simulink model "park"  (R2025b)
settings: Solver=FixedStepAuto  StartTime=0.0  StopTime=10.0  FixedStep=1e-4  RelTol=1e-3
undefined symbols (not defined in the file): DiscIntNeverNeededParam

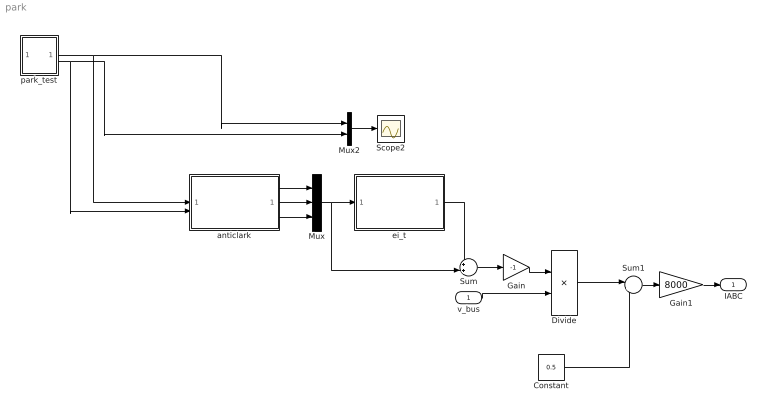
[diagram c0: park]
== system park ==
  v_bus : Inport
  Constant : Constant  Value=0.5
  Divide : Product  Inputs=*/
  Gain : Gain  Gain=-1
  Gain1 : Gain  Gain=8000
  Mux : Mux  Inputs=3
  Mux2 : Mux  Inputs=2
  Scope2 : Scope
  Sum : Sum  Inputs=++|
  Sum1 : Sum  Inputs=|++
  anticlark : Subsystem
  ei_t : Subsystem
  park_test : Subsystem
  IABC : Outport
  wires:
  Mux2/1 -> Scope2/1
  park_test/1(ualpha) -> anticlark/1(Valpha), Mux2/1
  park_test/2(ubeta) -> anticlark/2(Vbeta), Mux2/2
  anticlark/1(Va) -> Mux/1
  anticlark/2(Vb) -> Mux/2
  anticlark/3(Vc) -> Mux/3
  Mux/1 -> Sum/2, ei_t/1(Vabc)
  ei_t/1(ei_t1) -> Sum/1
  Sum/1 -> Gain/1
  Sum1/1 -> Gain1/1
  Gain1/1 -> IABC/1
  Gain/1 -> Divide/1
  v_bus/1 -> Divide/2
  Divide/1 -> Sum1/1
  Constant/1 -> Sum1/2

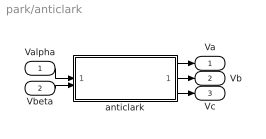
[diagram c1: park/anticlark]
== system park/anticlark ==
  Valpha : Inport
  Vbeta : Inport  Port=2
  anticlark : Subsystem
  Va : Outport
  Vb : Outport  Port=2
  Vc : Outport  Port=3
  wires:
  anticlark/3(Vc) -> Vc/1
  Vbeta/1 -> anticlark/2(Vbeta)
  anticlark/1(Va) -> Va/1
  anticlark/2(Vb) -> Vb/1
  Valpha/1 -> anticlark/1(Valpha)

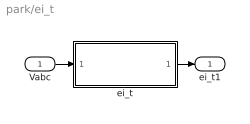
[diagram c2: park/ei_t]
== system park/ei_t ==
  Vabc : Inport
  ei_t : Subsystem
  ei_t1 : Outport
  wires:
  Vabc/1 -> ei_t/1(Vabc)
  ei_t/1(ei_t) -> ei_t1/1

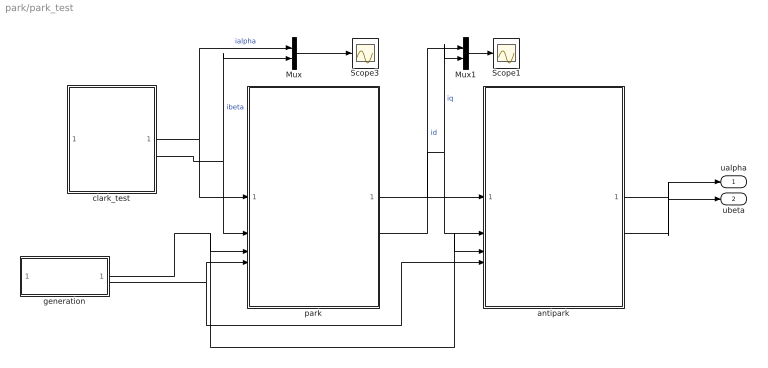
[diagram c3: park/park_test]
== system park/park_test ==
  Mux : Mux  Inputs=2
  Mux1 : Mux  Inputs=2
  Scope1 : Scope
  Scope3 : Scope
  antipark : Subsystem
  clark_test : Subsystem  TreatAsAtomicUnit=on
  generation : Subsystem
  park : Subsystem
  ualpha : Outport
  ubeta : Outport  Port=2
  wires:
  generation/2(cos) -> antipark/4(theta_cos), park/4(theta_cos)
  park/1(id) -> Mux1/1, antipark/1(ud)  "id"
  clark_test/1(ialpha) -> Mux/1, park/1(ialpha)  "ialpha"
  Mux1/1 -> Scope1/1
  clark_test/2(ibeta) -> Mux/2, park/2(ibeta)  "ibeta"
  generation/1(sin) -> antipark/3(theta_sin), park/3(theta_sin)
  park/2(iq) -> Mux1/2, antipark/2(uq)  "iq"
  Mux/1 -> Scope3/1
  antipark/2(ubeta) -> ubeta/1
  antipark/1(ualpha) -> ualpha/1

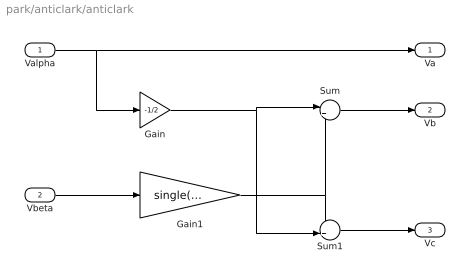
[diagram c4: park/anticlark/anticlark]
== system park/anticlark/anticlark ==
  Valpha : Inport
  Vbeta : Inport  Port=2
  Gain : Gain  Gain=-1/2
  Gain1 : Gain  Gain=single(sqrt(3)/2)
  Sum : Sum  Inputs=|++
  Sum1 : Sum  Inputs=-+|
  Va : Outport
  Vb : Outport  Port=2
  Vc : Outport  Port=3
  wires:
  Valpha/1 -> Gain/1, Va/1
  Gain/1 -> Sum1/2, Sum/1
  Gain1/1 -> Sum1/1, Sum/2
  Sum/1 -> Vb/1
  Vbeta/1 -> Gain1/1
  Sum1/1 -> Vc/1

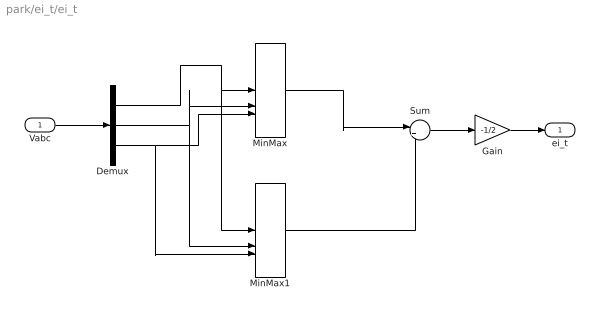
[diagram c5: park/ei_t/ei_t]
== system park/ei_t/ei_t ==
  Vabc : Inport
  Demux : Demux  Outputs=3
  Gain : Gain  Gain=-1/2
  MinMax : MinMax  Inputs=3
  MinMax1 : MinMax  Function=max  Inputs=3
  Sum : Sum  Inputs=|++
  ei_t : Outport
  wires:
  Vabc/1 -> Demux/1
  Demux/1 -> MinMax1/1, MinMax/1
  Demux/2 -> MinMax1/2, MinMax/2
  Demux/3 -> MinMax1/3, MinMax/3
  MinMax/1 -> Sum/1
  MinMax1/1 -> Sum/2
  Sum/1 -> Gain/1
  Gain/1 -> ei_t/1

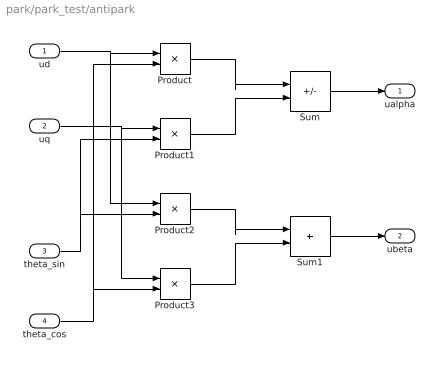
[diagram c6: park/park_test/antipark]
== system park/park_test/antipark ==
  ud : Inport
  uq : Inport  Port=2
  theta_sin : Inport  Port=3
  theta_cos : Inport  Port=4
  Product{,1..3} (4 alike) : Product
  Sum : Sum  Inputs=|+-
  Sum1 : Sum  Inputs=|++
  ualpha : Outport
  ubeta : Outport  Port=2
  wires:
  theta_cos/1 -> Product3/2, Product/2
  theta_sin/1 -> Product1/2, Product2/2
  uq/1 -> Product3/1, Product1/1
  ud/1 -> Product2/1, Product/1
  Product/1 -> Sum/1
  Product1/1 -> Sum/2
  Product2/1 -> Sum1/1
  Product3/1 -> Sum1/2
  Sum/1 -> ualpha/1
  Sum1/1 -> ubeta/1

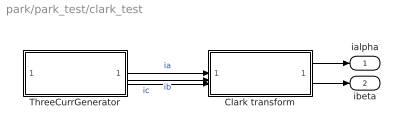
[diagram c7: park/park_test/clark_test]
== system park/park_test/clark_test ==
  Clark transform : Subsystem
  ThreeCurrGenerator : Subsystem
  ialpha : Outport
  ibeta : Outport  Port=2
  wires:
  Clark transform/1(ialpha) -> ialpha/1
  Clark transform/2(ibeta) -> ibeta/1
  ThreeCurrGenerator/1(ia) -> Clark transform/1(ia)  "ia"
  ThreeCurrGenerator/2(ib) -> Clark transform/2(ib)  "ib"
  ThreeCurrGenerator/3(ic) -> Clark transform/3(ic)  "ic"

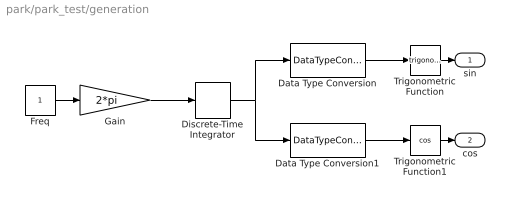
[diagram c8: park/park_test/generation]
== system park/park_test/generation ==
  Data Type Conversion : DataTypeConversion  OutDataTypeStr=single
  Data Type Conversion1 : DataTypeConversion  OutDataTypeStr=single
  Discrete-Time Integrator : DiscreteIntegrator  SampleTime=0.0001  ICPrevOutput=DiscIntNeverNeededParam  ICPrevScaledInput=DiscIntNeverNeededParam
  Freq : Constant
  Gain : Gain  Gain=2*pi
  Trigonometric Function : Trigonometry
  Trigonometric Function1 : Trigonometry  Operator=cos
  sin : Outport
  cos : Outport  Port=2
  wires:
  Freq/1 -> Gain/1
  Gain/1 -> Discrete-Time Integrator/1
  Discrete-Time Integrator/1 -> Data Type Conversion1/1, Data Type Conversion/1
  Data Type Conversion/1 -> Trigonometric Function/1
  Data Type Conversion1/1 -> Trigonometric Function1/1
  Trigonometric Function/1 -> sin/1
  Trigonometric Function1/1 -> cos/1

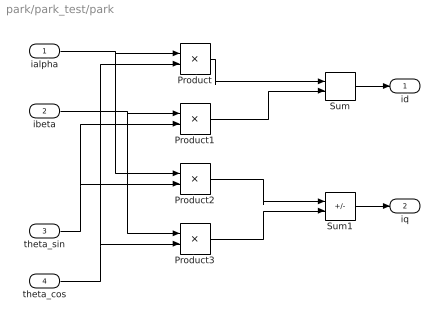
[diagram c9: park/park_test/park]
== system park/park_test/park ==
  ialpha : Inport
  ibeta : Inport  Port=2
  theta_sin : Inport  Port=3
  theta_cos : Inport  Port=4
  Product{,1..3} (4 alike) : Product
  Sum : Sum  Inputs=|++
  Sum1 : Sum  Inputs=|-+
  id : Outport
  iq : Outport  Port=2
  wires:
  ialpha/1 -> Product2/1, Product/1
  ibeta/1 -> Product1/1, Product3/1
  theta_sin/1 -> Product1/2, Product2/2
  theta_cos/1 -> Product3/2, Product/2
  Product/1 -> Sum/1
  Product1/1 -> Sum/2
  Product2/1 -> Sum1/1
  Product3/1 -> Sum1/2
  Sum1/1 -> iq/1
  Sum/1 -> id/1

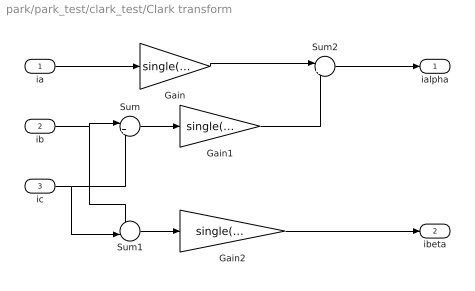
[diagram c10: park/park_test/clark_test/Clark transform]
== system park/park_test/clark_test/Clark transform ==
  ia : Inport
  ib : Inport  Port=2
  ic : Inport  Port=3
  Gain : Gain  Gain=single(2/3)
  Gain1 : Gain  Gain=single(1/3)
  Gain2 : Gain  Gain=single(sqrt(3)/3)
  Sum : Sum  Inputs=|++
  Sum1 : Sum  Inputs=+-|
  Sum2 : Sum  Inputs=|+-
  ialpha : Outport
  ibeta : Outport  Port=2
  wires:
  ia/1 -> Gain/1
  ib/1 -> Sum1/1, Sum/1
  ic/1 -> Sum1/2, Sum/2
  Sum/1 -> Gain1/1
  Sum1/1 -> Gain2/1
  Gain/1 -> Sum2/1
  Gain1/1 -> Sum2/2
  Gain2/1 -> ibeta/1
  Sum2/1 -> ialpha/1

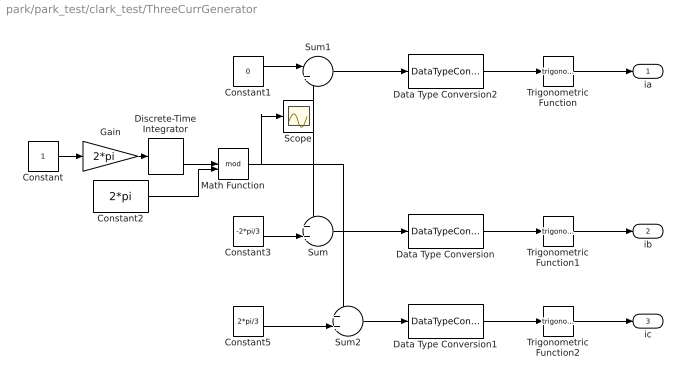
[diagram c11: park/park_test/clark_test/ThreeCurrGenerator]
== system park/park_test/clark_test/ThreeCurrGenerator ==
  Constant : Constant
  Constant1 : Constant  Value=0
  Constant2 : Constant  Value=2*pi
  Constant3 : Constant  Value=-2*pi/3
  Constant5 : Constant  Value=2*pi/3
  Data Type Conversion : DataTypeConversion  OutDataTypeStr=single
  Data Type Conversion1 : DataTypeConversion  OutDataTypeStr=single
  Data Type Conversion2 : DataTypeConversion  OutDataTypeStr=single
  Discrete-Time Integrator : DiscreteIntegrator  SampleTime=0.0001  ICPrevOutput=DiscIntNeverNeededParam  ICPrevScaledInput=DiscIntNeverNeededParam
  Gain : Gain  Gain=2*pi
  Math Function : Math  Operator=mod
  Scope : Scope
  Sum : Sum  Inputs=++|
  Sum1 : Sum  Inputs=|++
  Sum2 : Sum  Inputs=++|
  Trigonometric Function : Trigonometry
  Trigonometric Function1 : Trigonometry
  Trigonometric Function2 : Trigonometry
  ia : Outport
  ib : Outport  Port=2
  ic : Outport  Port=3
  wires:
  Constant/1 -> Gain/1
  Gain/1 -> Discrete-Time Integrator/1
  Constant3/1 -> Sum/2
  Constant1/1 -> Sum1/1
  Sum1/1 -> Data Type Conversion2/1
  Sum/1 -> Data Type Conversion/1
  Sum2/1 -> Data Type Conversion1/1
  Constant5/1 -> Sum2/2
  Data Type Conversion2/1 -> Trigonometric Function/1
  Trigonometric Function/1 -> ia/1
  Data Type Conversion/1 -> Trigonometric Function1/1
  Trigonometric Function1/1 -> ib/1
  Data Type Conversion1/1 -> Trigonometric Function2/1
  Trigonometric Function2/1 -> ic/1
  Discrete-Time Integrator/1 -> Math Function/1
  Constant2/1 -> Math Function/2
  Math Function/1 -> Sum2/1, Sum1/2, Sum/1, Scope/1
